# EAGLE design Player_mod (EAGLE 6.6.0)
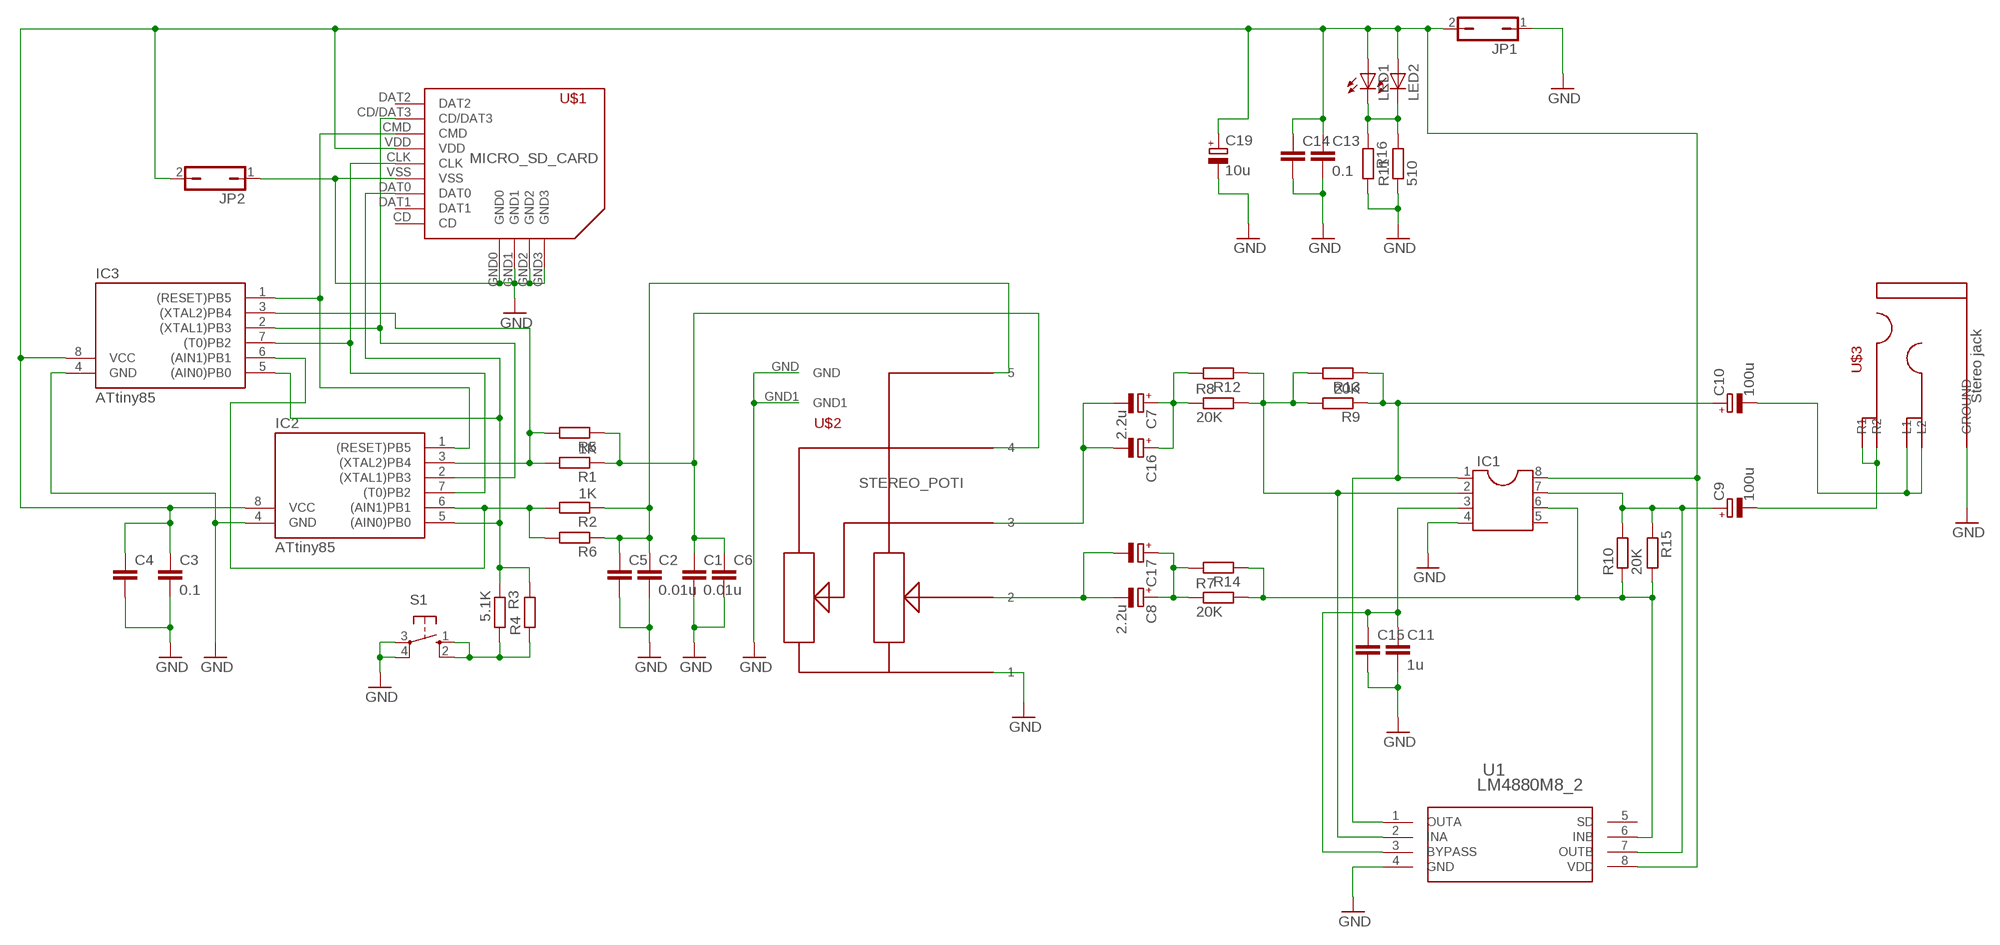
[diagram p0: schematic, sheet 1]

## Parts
C1  0.01u  C-EUC2012  [C2012]
C2  0.01u  C-EUC2012  [C2012]
C3  0.1  C-EUC2012  [C2012]
C4  C-EU050-025X075  [C050-025X075]
C5  C-EU050-025X075  [C050-025X075]
C6  C-EU050-025X075  [C050-025X075]
C7  2.2u  CPOL-EU085CS-1AR  [085CS_1AR]
C8  2.2u  CPOL-EU085CS-1AR  [085CS_1AR]
C9  100u  CPOL-EUE5-8.5  [E5-8,5]
C10  100u  CPOL-EUE5-8.5  [E5-8,5]
C11  1u  C-EUC2012  [C2012]
C13  0.1  C-EUC2012  [C2012]
C14  C-EU050-025X075  [C050-025X075]
C15  C-EU050-025X075  [C050-025X075]
C16  CPOL-EUE2.5-6  [E2,5-6]
C17  CPOL-EUE2.5-6  [E2,5-6]
C19  10u  CPOL-EUE5-8.5  [E5-8,5]
IC1  DIL8  [DIL08]
IC2  ATtiny85  TINY10P  [DIL08]
IC3  ATtiny85  TINY10S  [SOIC8]
JP1  JP1Q  [JP1]
JP2  JP1Q  [JP1]
LED1  LED5MM  [LED5MM]
LED2  LEDCHIPLED_0805  [CHIPLED_0805]
R1  1K  R-EU_R2012  [R2012]
R2  1K  R-EU_R2012  [R2012]
R3  5.1K  R-EU_R2012  [R2012]
R4  R-EU_0204/7  [0204/7]
R5  R-EU_0204/7  [0204/7]
R6  R-EU_0204/7  [0204/7]
R7  20K  R-EU_R2012  [R2012]
R8  20K  R-EU_R2012  [R2012]
R9  20K  R-EU_R2012  [R2012]
R10  20K  R-EU_R2012  [R2012]
R11  510  R-EU_R2012  [R2012]
R12  R-EU_0204/7  [0204/7]
R13  R-EU_0204/7  [0204/7]
R14  R-EU_0204/7  [0204/7]
R15  R-EU_0204/7  [0204/7]
R16  R-EU_0204/7  [0204/7]
S1  10-XX  [B3F-10XX]
U1  LM4880M8_2  [SO8NB]
U$1  MICRO_SD_CARD  [MICRO_SD_CARD]
U$2  STEREO_POTI  [STEREO_POTI]
U$3  STEREO_JACK  [STEREO_JACK]

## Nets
GND: C1.2 C2.2 C3.2 C4.2 C5.2 C6.2 C11.2 C13.2 C14.2 C15.2 C19.- IC1.4 IC2.4(GND) IC3.4(GND) JP1.1 JP2.1 R11.1 R16.2 S1.3(P) S1.4(P1) U1.4(GND) U$1.GND0 U$1.GND1 U$1.GND2 U$1.GND3 U$1.VSS U$2.1 U$2.GND U$2.GND1 U$3.GROUND
N$1: C1.1 C6.1 R1.1 R5.1 U$2.4
N$2: C3.1 C4.1 C13.1 C14.1 C19.+ IC1.8 IC2.8(VCC) IC3.8(VCC) JP1.2 JP2.2 LED1.A LED2.A U1.8(VDD) U$1.VDD
N$3: C8.- C17.- U$2.2
N$4: IC2.6((AIN1)PB1) IC3.6((AIN1)PB1) R2.2 R6.2
N$5: C2.1 C5.1 R2.1 R6.1 U$2.5
N$6: IC2.5((AIN0)PB0) IC3.5((AIN0)PB0) R3.1 R4.2 U$1.DAT0
N$7: IC2.3((XTAL2)PB4) IC3.3((XTAL2)PB4) R1.2 R5.2
N$8: C7.- C16.- U$2.3
N$9: R3.2 R4.1 S1.1(S) S1.2(S1)
N$10: C10.- U$3.L1 U$3.L2
N$11: C9.- U$3.R1 U$3.R2
N$12: IC2.7((T0)PB2) IC3.7((T0)PB2) U$1.CLK
N$15: C11.1 C15.1 IC1.3 U1.3(BYPASS)
N$16: IC2.1((RESET)PB5) IC3.1((RESET)PB5) U$1.CMD
N$17: C8.+ C17.+ R7.1 R14.2
N$18: IC2.2((XTAL1)PB3) IC3.2((XTAL1)PB3) U$1.CD/DAT3
N$19: C7.+ C16.+ R8.1 R12.2
N$20: IC1.2 R8.2 R9.2 R12.1 R13.2 U1.2(INA)
N$22: C10.+ IC1.1 R9.1 R13.1 U1.1(OUTA)
N$23: C9.+ IC1.7 R10.2 R15.1 U1.7(OUTB)
N$24: LED1.K(C) LED2.C R11.2 R16.1
N$29: IC1.6 R7.2 R10.1 R14.1 R15.2 U1.6(INB)
Unconnected: IC1.5 U1.5(SD) U$1.CD U$1.DAT1 U$1.DAT2

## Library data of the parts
C1-C6 C11 C13-C15 = rcl:C-EU: CAPACITOR, European symbol
C7-C10 C16 C17 C19 = rcl:CPOL-EU: POLARIZED CAPACITOR, European symbol
IC1 = ic-package:DIL8: Dual In Line / Socket
IC2 IC3 = atmel:TINY10: MICROCONTROLLER 1 Kbytes ROM; OC_FARNELL: unknown; OC_NEWARK: unknown
JP1 JP2 = jumper:JP1Q: JUMPER
LED1 LED2 = led:LED: LED
R1-R4 R7-R16 = rcl:R-EU_: RESISTOR, European symbol
R5 R6 = resistor:R-EU_: RESISTOR, European symbol
S1 = switch-omron:10-XX: OMRON SWITCH
U1 = LM4880M:LM4880M8_2; DATABASE: INTEGRATEDCIRCUITS; FOOTPRINT_NAME: SO8; ID: 151511; MANUFACTURER_PART_NUMBER: LM4880M8_2; ORIGINALNAME: LM4880M8_2; VENDOR: NSC
U$1 = Micro_SD_card_connector:MICRO_SD_CARD: Micro SD card connector
U$2 = STEREO_POTI:STEREO_POTI: Stereo potentiometer with wheel
U$3 = Player:STEREO_JACK

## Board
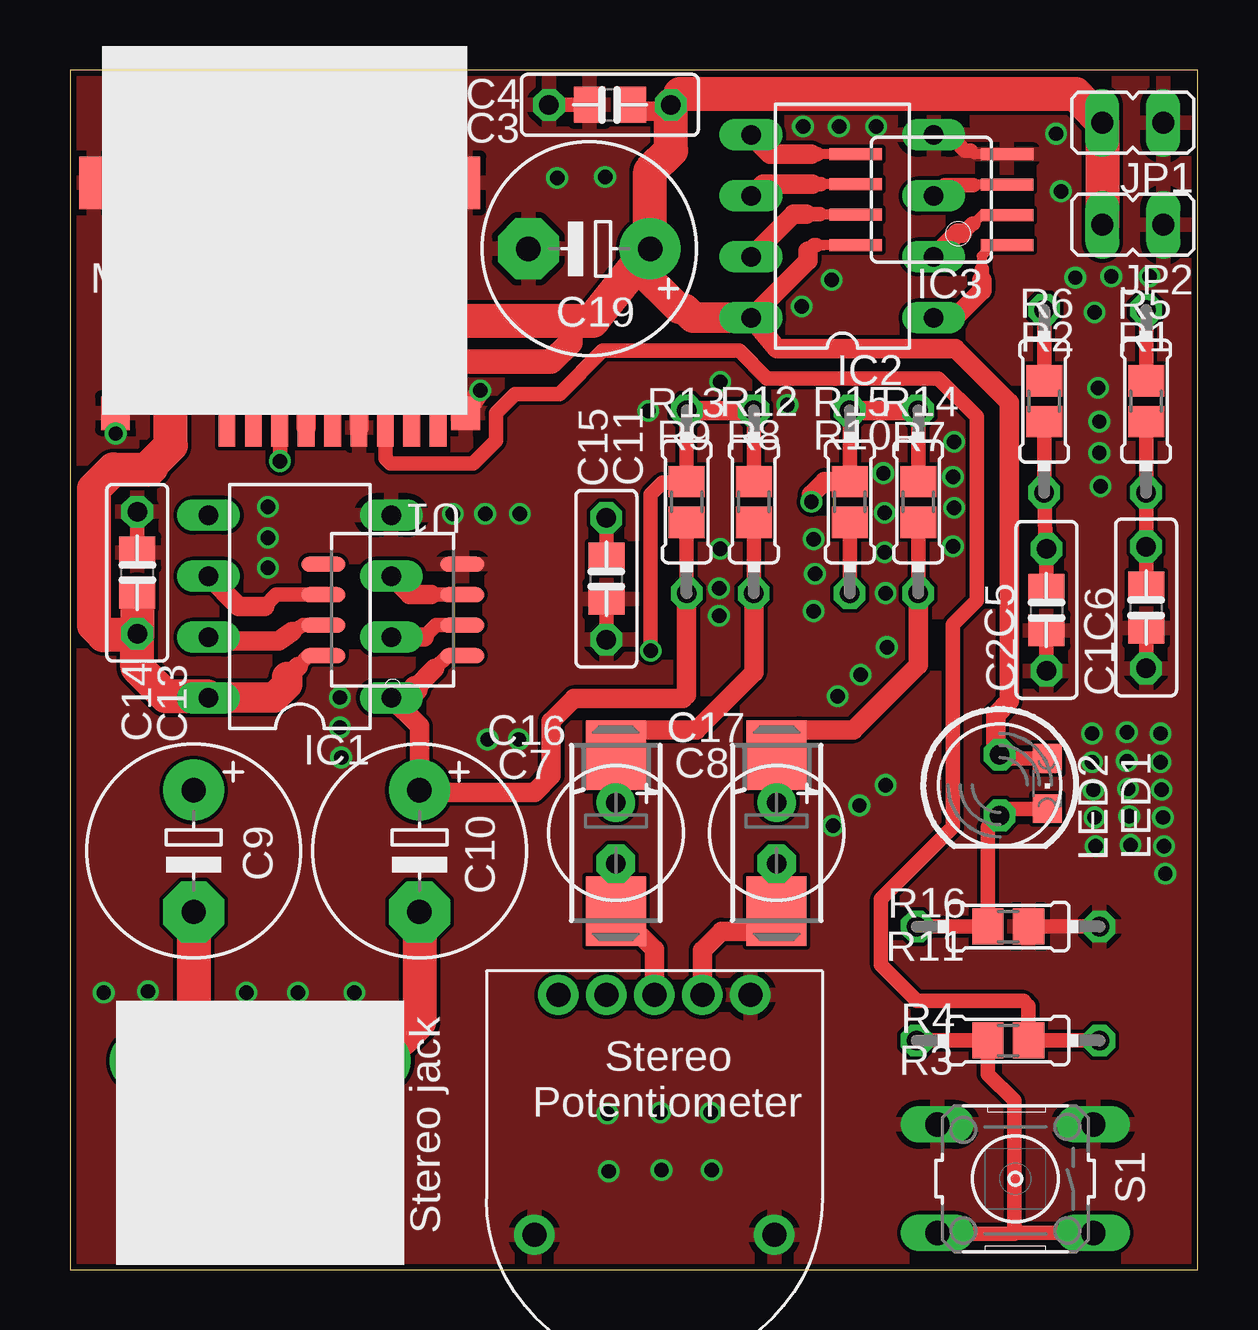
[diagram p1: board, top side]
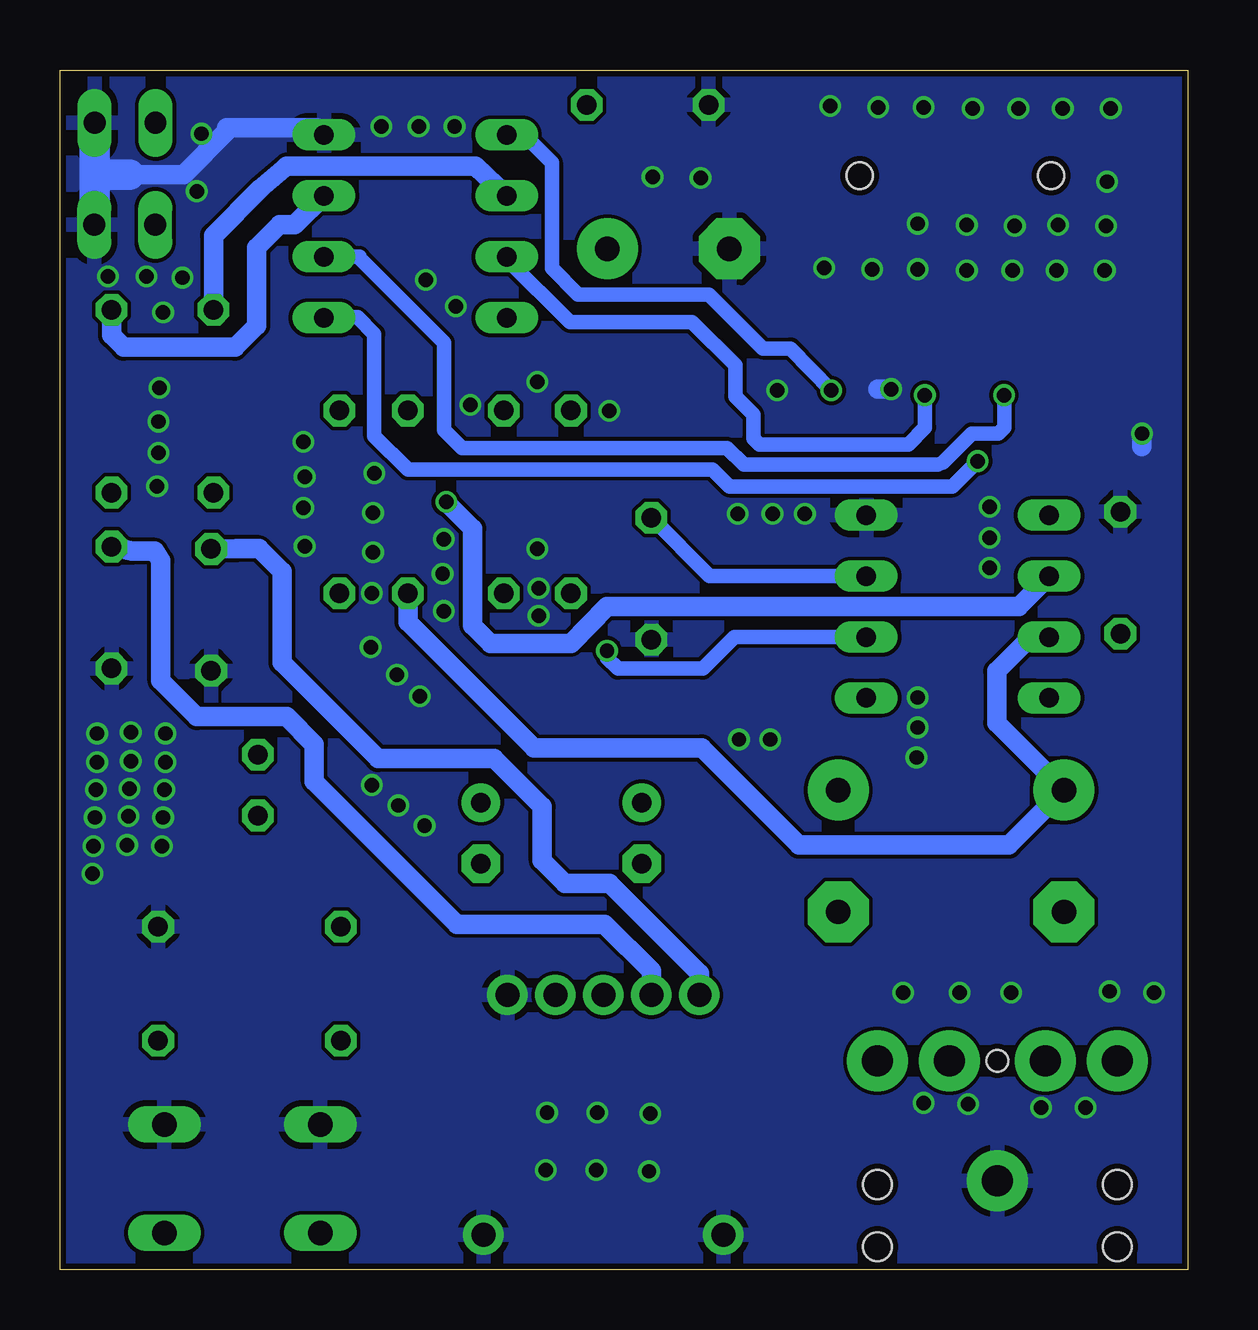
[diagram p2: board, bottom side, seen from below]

Size 47 x 50 mm. Coordinates in mm from the lower left corner, seen from the top.
Outline: 0,0 47,0 47,50 0,50 0,0
Copper layers (1*16): Top 0.035mm / dielectric 1.5mm / Bottom 0.035mm
Design rules "ITEADstudio_DRC": minimum track width 6mil, minimum drill 12mil, track to track 6mil, track to pad 6mil, pad to pad 6mil, via to via 6mil, smd to smd 0mil, copper to edge 10mil, drill to drill 10mil, minimum pad ring 10mil, minimum via ring 6mil, stop-mask expansion 2mil, vias tented up to drill 100mil, thermal gap 10mil

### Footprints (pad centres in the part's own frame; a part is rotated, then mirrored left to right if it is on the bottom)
C2012 = smd 1.3 x 1.5: 1 -0.85,0; 2 0.85,0
C050-025X075 = drill 0.813 octagon: 1 -2.54,0; 2 2.54,0
085CS_1AR = smd 2.9 x 2.5: + 3.25,0; - -3.25,0
E5-8,5 = drill 1.016 pad 2.54: + -2.54,0 | drill 1.016 pad 2.54 octagon: - 2.54,0
E2,5-6 = drill 0.813 pad 1.6: + -1.27,0 | drill 0.813 pad 1.6 octagon: - 1.27,0
DIL08 = drill 0.813 long: 1 -3.81,-3.81; 2 -1.27,-3.81; 3 1.27,-3.81; 4 3.81,-3.81; 5 3.81,3.81; 6 1.27,3.81; 7 -1.27,3.81; 8 -3.81,3.81
SOIC8 = smd 0.5 x 2.2: 1 -1.905,-3.154; 2 -0.645,-3.154; 3 0.625,-3.154; 4 1.895,-3.154; 5 1.905,3.154; 6 0.635,3.154; 7 -0.635,3.154; 8 -1.905,3.154
JP1 = drill 0.914 long: 1 0,-1.27; 2 0,1.27
LED5MM = drill 0.813 octagon: A -1.27,0; K 1.27,0
CHIPLED_0805 = smd 1.2 x 1.2: A 0,-1.05; C 0,1.05
R2012 = smd 1.3 x 1.5: 1 -0.85,0; 2 0.85,0
0204/7 = drill 0.813 octagon: 1 -3.81,0; 2 3.81,0
B3F-10XX = drill 1.016 long: 1 -3.251,2.261; 2 3.251,2.261; 3 -3.251,-2.261; 4 3.251,-2.261
SO8NB = smd 1.829 x 0.635: 1 -2.896,1.905; 2 -2.896,0.635; 3 -2.896,-0.635; 4 -2.896,-1.905; 5 2.896,-1.905; 6 2.896,-0.635; 7 2.896,0.635; 8 2.896,1.905
MICRO_SD_CARD = smd 0.7 x 1.6: CD -6.6,5.6; CD/DAT3 1.1,5.6; CLK -2.2,5.6; CMD 0,5.6; DAT0 -4.4,5.6; DAT1 -5.5,5.6; DAT2 2.2,5.6; VDD -1.1,5.6; VSS -3.3,5.6 | smd 1.2 x 1.4: GND0 -7.75,5; GND3 6.85,5 | smd 1.2 x 2.2: GND1 -7.75,-4.6; GND2 7.75,-4.6 | hole 1.1: -4.93,-4.9; 3.05,-4.9
STEREO_POTI = drill 1 pad 1.676: 1 0,4; 2 0,2; 3 0,0; 4 0,-2; 5 0,-4; GND 10,5; GND1 10,-5
STEREO_JACK = drill 1.3 pad 2.54: GROUND -2,0; L1 3,-2; L2 3,-5; R1 3,5; R2 3,2 | hole 1.2: -2.15,-5; -2.15,5; -4.75,-5; -4.75,5 | hole 0.9: 3,0

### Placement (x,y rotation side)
C1  44.85,27.6 270 top
C2  40.7,27.5 270 top
C3  22.5,48.55 180 top
C4  22.5,48.55 180 top
C5  40.7,27.5 270 top
C6  44.85,27.6 270 top
C7  22.75,18.2 90 top
C8  29.45,18.2 90 top
C9  5.15,17.45 270 top
C10  14.56,17.45 270 top
C11  22.35,28.8 270 top
C13  2.8,29.05 90 top
C14  2.8,29.05 90 top
C15  22.35,28.8 270 top
C16  22.75,18.2 270 top
C17  29.45,18.2 270 top
C19  21.64,42.55 180 top
IC1  9.58,27.64 90 top
IC2  32.19,43.49 90 top
IC3  35.9,44.6 90 top
JP1  44.29,47.8 90 top
JP2  44.3,43.55 90 top
LED1  38.75,20.2 270 top
LED2  40.73,20.26 180 top
R1  44.85,36.2 90 top
R2  40.6,36.2 90 top
R3  39.1,9.55 180 top
R4  39.1,9.55 0 top
R5  44.85,36.2 90 top
R6  40.6,36.2 90 top
R7  35.35,32 90 top
R8  28.5,32 90 top
R9  25.7,32 90 top
R10  32.5,32 270 top
R11  39.1,14.3 180 top
R12  28.5,32 270 top
R13  25.7,32 90 top
R14  35.35,32 270 top
R15  32.5,32 90 top
R16  39.1,14.3 0 top
S1  39.4,3.79 180 top
U1  13.45,27.5 180 top
U$1  8.74,40.7 180 top
U$2  24.35,11.45 270 top
U$3  7.93,5.7 90 top

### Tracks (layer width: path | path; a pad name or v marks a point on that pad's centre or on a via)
GND  (via drill 0.6)
  Top 0.406: IC3.4 37.7,46.49 37.55,46.65
  Top 0.61: C4.2 C3.2 | C13.2 C14.2 | C15.2 C11.2 | R11.1 R16.2 | C5.2 C2.2 | C1.2 C6.2 | 37.55,46.65 37.3,46.65 36.85,47.1 36.2,47.1 IC2.4
  Top 0.813: U$1.GND3 v1.89,34.86 v1.9,34.85 | U$1.VSS 12.04,36.39 v12.35,36.7 | U$1.GND0 v17.1,36.65
  Bottom 0.61: 45.55,48.39 JP1.1
  Bottom 0.813: v1.9,34.85 1.9,34.3 | v12.35,36.7 12.9,36.7 | IC2.4 36.3,47.6 40.05,47.6 40.05,47.45 41.85,45.65 44.1,45.65
  Bottom 1.27: 45.55,43.45 45.55,45.65 | 45.55,45.65 45.55,48.39 | 44.1,45.65 45.55,45.65
  other vias: 30.55,47.65 32.05,47.65 33.6,47.65 11.25,43.6 30.5,40.15 9.2,43.55 5.4,43.55 41.9,41.35 7.2,43.5 3.35,45.35 31.75,41.25 3.4,43.5 27.1,37 34.05,25.95 27.1,30.05 27.05,28.4 24.1,35.8 29.9,36.05 31.05,29 31,27.45 31,30.45 27.05,27.25 33.9,33.2 33.95,31.55 33.95,29.9 34,28.2 36.85,34.5 36.8,33.05 36.85,31.75 36.8,30.15 45.45,22.35 45.45,21.15 45.5,20 45.55,18.85 45.6,17.65 45.65,16.5 44.05,22.4 44.05,21.2 44.1,20.05 44.15,18.9 44.2,17.7 42.6,22.35 42.6,21.15 42.65,20 42.7,18.85 42.75,17.65 31.8,18.5 32.9,19.35 34,20.2 8.25,31.8 8.25,30.5 8.25,29.25 11.3,21.35 11.25,23.85 11.25,22.6 3.2,48.4 5.2,48.4 7.05,48.4 8.95,48.4 11,48.45 12.9,48.45 14.9,48.5 3.45,41.65 5.45,41.65 7.3,41.65 9.2,41.65 11.25,41.7 13.15,41.7 15.15,41.75 11,6.95 9.5,11.55 11.85,11.55 4.25,6.75 6.1,6.75 9.15,6.9 22.4,6.5 24.6,6.55 26.7,6.55 22.45,4.1 24.65,4.15 26.75,4.15 20.3,45.5 22.3,45.55 7.35,11.55 1.4,11.55 3.25,11.6 43.4,41.4 45,41.4 42.9,35.35 42.9,34.05 42.95,32.65 41.1,47.35 42.7,39.9 41.3,44.95 42.85,36.75 32.95,24.8 32,23.9 18.7,22.1 17.4,22.1 15.95,31.5 17.3,31.5 18.75,31.5
  pour Bottom: 0,51 48,51 48,-1 0,-1
  pour Top: 0,50 47,50 47,0 0,0
N$1
  Top 0.61: C1.1 C6.1 R5.1 R1.1
  Bottom 0.813: U$2.4 22.35,12.45 24.3,14.4 30.45,14.4 36.4,20.35 36.4,21.9 37.55,23.05 41.3,23.05 42.8,24.55 42.8,29.55 43.05,29.95 44.01,29.95 C6.1
N$2
  Top 0.406: IC3.8 31.41,42.7 31.4,42.7 31.1,42.7
  Top 0.61: LED2.A 38.91,21.31 LED1.A | 23.6,41.82 23.6,41.97 C19.+ | 31.1,42.7 31,42.7 30.75,42.45 | U1.8 9.95,25.59 9.5,25.15
  Top 0.813: LED1.A 38.58,21.47 38.58,23.13 39.15,23.7 39.15,36.15 36.9,38.4 29.46,38.4 IC2.8 30.75,42.05 30.75,42.45 | U$1.VDD 9.84,36.99 9.85,37 9.85,37.05 | 24.78,48.29 23.35,48.29 C3.1 | C4.1 25.44,48.55 25.44,49 | 9.5,25.15 9.05,24.7
  Top 1.016: 24.78,48.29 C4.1 | 9.85,37.05 9.95,37.05 10.75,37.85 20.05,37.85 20.85,38.65 20.85,39.4 20.7,39.55
  Top 1.27: 5.7,23.9 IC1.8 5.79,23.85 8.5,23.85 9.05,24.4 9.05,24.7 | IC2.8 25.97,39.68 25.6,40.05 25.37,40.05 23.6,41.82
  Top 1.422: 25.44,49 41.92,49 JP1.2 JP2.2 | 5.7,23.9 4,23.9 2.8,25.1 2.8,26.45 | 2.8,26.45 C14.1 C13.1 | 2.8,26.45 1.4,26.45 1,26.85 1,32.55 1.8,33.35 3.3,33.35 3.4,33.45 3.4,33.55 4.2,34.35 4.2,37.7 6.05,39.55 20.7,39.55 21.78,39.55 C19.+ 24.18,45.78 25.05,46.65 C4.1
N$3
  Top 0.61: C17.- C8.-
  Top 0.813: U$2.2 26.35,13.3 27.15,14.1 28.6,14.1 C8.-
N$4
  Top 0.406: IC3.6 31.32,45.23 31.3,45.25
  Top 0.61: R2.2 R6.2 | 31.3,45.25 30.95,45.25
  Top 0.813: 30.95,45.25 28.87,45.25 IC2.6
  Bottom 0.813: IC2.6 29.67,46 37.55,46 38.65,45.05 40.6,43.1 R6.2
N$5
  Top 0.61: C2.1 C5.1 40.65,30.49 R6.1 R2.1
  Bottom 0.813: U$2.5 20.35,12.35 24.1,16.1 25.95,16.1 26.9,17.05 26.9,19.3 28.9,21.3 33.75,21.3 37.75,25.3 37.75,29.1 38.7,30.05 39.64,30.05 C5.1
N$6  (via drill 0.6)
  Top 0.406: IC3.5 31.15,46.51 31.15,46.5
  Top 0.61: R4.2 R3.1 39.95,11 39.75,11.2 35.3,11.2 33.8,12.7 33.8,15.45 36.8,18.45 36.8,26.9 37.8,27.9 37.8,35.55 36.2,37.15 29.05,37.15 27.9,38.3 22.2,38.3 20.4,36.5 18.55,36.5 17.75,35.7 17.75,34.55 16.8,33.6 13.35,33.6 13.15,33.8 U$1.DAT0 13.15,35.95 13.75,36.65 v14.85,36.65 | 31.15,46.5 30.9,46.5
  Top 0.813: 30.9,46.5 29.18,46.5 IC2.5
  Bottom 0.61: IC2.5 27.65,47.3 26.5,46.15 26.5,41.75 25.4,40.65 19.95,40.65 17.7,38.4 16.55,38.4 v14.85,36.65
N$7
  Top 0.406: IC3.3 37.67,45.23 37.65,45.2
  Top 0.61: R1.2 R5.2 | 37.65,45.2 36.44,45.2 IC2.3
  Bottom 0.813: IC2.3 37.21,43.55 37.85,43.55 38.8,42.6 38.8,39.35 39.7,38.45 44.35,38.45 44.85,38.95 R5.2
N$8
  Top 0.61: C16.- C7.-
  Top 0.813: U$2.3 24.35,13.35 C7.-
N$9
  Top 0.61: R4.1 R3.2 38.25,8.15 39.35,7.05 39.35,1.75 | 39.35,1.75 39.35,1.5 36.18,1.5 S1.2 | S1.1 39.57,1.53 39.35,1.75
N$10
  Top 1.422: C10.- 14.56,10.33 U$3.L2 U$3.L1
N$11
  Top 1.422: C9.- 5.15,8.7 U$3.R2 U$3.R1
N$12  (via drill 0.6)
  Top 0.406: IC3.7 31.29,43.97 31.25,44
  Top 0.61: v10.95,36.45 U$1.CLK | 31.25,44 30.7,44
  Top 0.813: 30.7,44 30.16,44 IC2.7
  Bottom 0.61: IC2.7 28.38,42.13 25.75,39.5 20.65,39.5 18.85,37.7 18.85,36.4 18.1,35.65 18.1,34.65 17.85,34.4 11.64,34.4 U$1.CLK v10.94,36.44 v10.95,36.45
N$15
  Top 0.61: C11.1 C15.1 | U1.3 15.06,28.14 15.05,28.15
  Top 0.813: 15.05,28.15 14.15,28.15 IC1.3
  Bottom 0.61: IC1.3 19.92,28.91 C15.1
N$16  (via drill 0.6)
  Top 0.406: IC3.1 38.45,42.7 38,42.25 38,41.7
  Top 0.61: v8.75,33.7 U$1.CMD | 38,41.7 38,41.25
  Top 0.813: 38,41.25 38,40.8 36.9,39.7 36.02,39.7 IC2.1
  Bottom 0.61: 9,33.45 v8.75,33.7 9.8,32.65 19.1,32.65 19.8,33.35 32.5,33.35 33.9,34.75 33.9,39 34.6,39.7 35.98,39.7 IC2.1
N$17
  Top 0.61: R7.1 R14.2 | C17.+ C8.+
  Top 0.813: R14.2 35.35,25.2 32.65,22.5 30.4,22.5 29.45,21.55 C8.+
N$18  (via drill 0.6)
  Top 0.406: IC3.2 38.01,43.95 37.65,43.6
  Top 0.61: v7.65,36.45 U$1.CD/DAT3 | 37.65,43.6 37.6,43.6 37.2,43.2
  Top 0.813: 37.2,43.2 36.98,43.2 IC2.2
  Bottom 0.61: IC2.2 34.52,42.22 34.52,42.17 31,38.65 31,35 30.25,34.25 19.2,34.25 18.5,33.55 10.4,33.55 10.2,33.65 9,34.85 7.89,34.85 U$1.CD/DAT3 v7.64,36.44 v7.65,36.45
N$19
  Top 0.61: R12.2 R8.1
  Top 0.813: C16.+ C7.+ 23.8,22.5 26.1,22.5 28.5,24.9 R12.2
N$20  (via drill 0.6)
  Top 0.61: R8.2 R12.1 | R13.2 R9.2 25.65,32.8 24.7,32.8 24.2,32.3 v24.2,25.8 | U1.2 15.24,26.86 14.75,26.37
  Top 0.813: R12.1 R13.2 | 14.75,26.37 IC1.2
  Bottom 0.61: IC1.2 18.88,26.37 20.2,25.05 23.75,25.05 24.2,25.5 v24.2,25.8
N$22
  Top 0.61: R9.1 R13.1 | U1.1 15.74,25.59 15.2,25.05
  Top 0.813: IC1.1 14.56,22.66 C10.+ 14.65,19.9 19.35,19.9 20.05,20.6 20.05,22.85 21,23.8 25.55,23.8 25.7,23.95 R13.1 | 15.2,25.05 14.4,24.25
  Top 1.016: 14.4,24.25 14.4,24.2 14,23.8 13.42,23.8 IC1.1
N$23
  Top 0.61: R10.2 R15.1 | U1.7 9.71,26.86 9.25,26.6
  Top 0.813: 9.25,26.6 8.7,26.2 5.94,26.2 IC1.7
  Bottom 0.152: IC1.7 6.35,26.67 6.55,26.35
  Bottom 0.813: R15.1 32.5,27 27.25,21.75 20.25,21.75 16.2,17.7 7.44,17.7 C9.+ 7.95,22.79 7.95,24.95 6.55,26.35 5.79,26.35
N$24
  Top 0.61: R16.1 R11.2 38.25,18.45 39.01,19.21 LED2.C 39.03,19.21 LED1.K
N$29  (via drill 0.6)
  Top 0.61: R15.2 R10.1 | R14.1 R7.2 | U1.6 8.59,28.14 8.1,27.65
  Top 0.813: R14.1 R15.2 | v30.9,32 30.9,32.3 31.45,32.85 R10.1 | 8.1,27.65 7.03,27.65 IC1.6
  Bottom 0.813: IC1.6 7.03,27.65 24.2,27.65 25.7,26.1 29.05,26.1 29.8,26.85 29.8,30.9 v30.9,32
